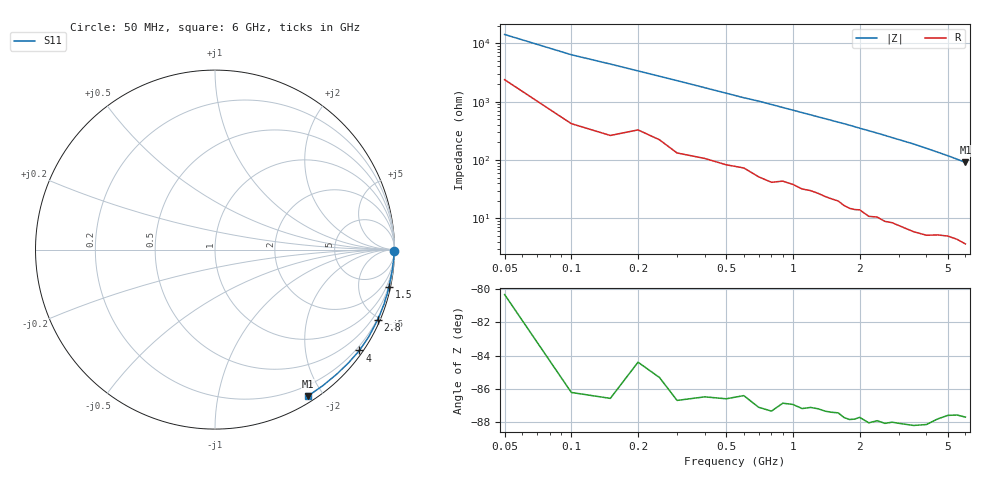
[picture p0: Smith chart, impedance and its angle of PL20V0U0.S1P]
! Infineon Technologies  Discrete & RF Semiconductors
! BAR 64-04W /-05W /-06W
! Si PIN Diode in SOT323
! VR = 20 V
! S-Parameters:  October  2008
# GHz  S  MA  R  50
!  f  S11
! GHz  MAG  ANG
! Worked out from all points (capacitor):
!   34 points, 50 MHz to 6 GHz, reference 50 ohm
!   read as one part to ground: C = 242 fF near 50 MHz
!   lowest |Z| = 90.9 ohm at 6 GHz (marker M1)
!   S11 on the Smith chart (normalised r, x): 50 MHz: open; 1.5 GHz: 0.43, -9.50; 2.8 GHz: 0.17, -4.84; 4 GHz: 0.10, -3.18; 6 GHz: 0.07, -1.82
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0.05  0.9988 -0.4
0.1  0.999 -0.9
0.15  0.9986 -1.3
0.2  0.9971 -1.7
0.3  0.9975 -2.5
0.5  0.9958 -4.1
0.6  0.9946 -4.9
0.7  0.9951 -5.6
0.8  0.9948 -6.4
0.9  0.9931 -7.2
1.1  0.9925 -8.8
1.5  0.9906 -12.0
1.6  0.9901 -12.8
1.7  0.9907 -13.6
1.8  0.9907 -14.4
1.9  0.99 -15.3
2  0.9889 -16.2
2.2  0.9895 -17.9
2.4  0.9878 -19.6
2.6  0.9878 -21.4
2.8  0.9863 -23.3
3  0.9858 -25.1
3.5  0.9845 -29.7
4  0.9816 -34.9
4.5  0.9755 -40.3
5  0.9703 -45.7
5.5  0.9673 -51.5
6  0.9665 -57.6
